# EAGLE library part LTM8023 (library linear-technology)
2A, 36V DC/DC µModule Complete Step-Down Switch Mode Power Supply Source: http://www.linear.com/pc/downloadDocument.do?name=8023ff.pdf
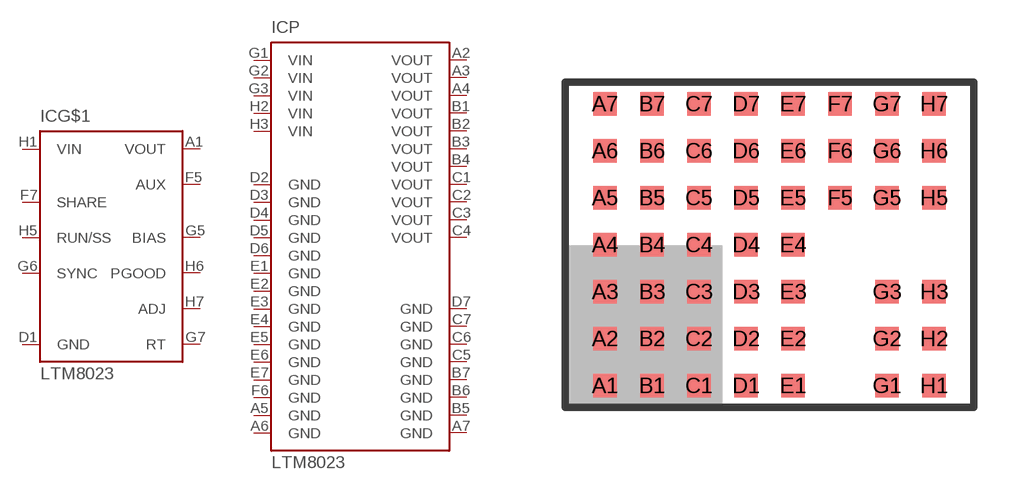
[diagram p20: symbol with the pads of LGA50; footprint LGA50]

Designator prefix IC; gates G$1=LTM8023 P=LTM8023-P

## LTM8023 (MPN: LTM8023IV#PBF; OC_FARNELL: 1799827; OC_NEWARK: 02P7640)  [LGA50]
A1  G$1:VOUT  pwr
A2  P:VOUT  pwr
A3  P:VOUT  pwr
A4  P:VOUT  pwr
A5  P:GND  pwr
A6  P:GND  pwr
A7  P:GND  pwr
B1  P:VOUT  pwr
B2  P:VOUT  pwr
B3  P:VOUT  pwr
B4  P:VOUT  pwr
B5  P:GND  pwr
B6  P:GND  pwr
B7  P:GND  pwr
C1  P:VOUT  pwr
C2  P:VOUT  pwr
C3  P:VOUT  pwr
C4  P:VOUT  pwr
C5  P:GND  pwr
C6  P:GND  pwr
C7  P:GND  pwr
D1  G$1:GND  pwr
D2  P:GND  pwr
D3  P:GND  pwr
D4  P:GND  pwr
D5  P:GND  pwr
D6  P:GND  pwr
D7  P:GND  pwr
E1  P:GND  pwr
E2  P:GND  pwr
E3  P:GND  pwr
E4  P:GND  pwr
E5  P:GND  pwr
E6  P:GND  pwr
E7  P:GND  pwr
F5  G$1:AUX  out
F6  P:GND  pwr
F7  G$1:SHARE  in
G1  P:VIN  pwr
G2  P:VIN  pwr
G3  P:VIN  pwr
G5  G$1:BIAS  pas
G6  G$1:SYNC  in
G7  G$1:RT  pas
H1  G$1:VIN  pwr
H2  P:VIN  pwr
H3  P:VIN  pwr
H5  G$1:RUN/SS  in
H6  G$1:PGOOD  oc
H7  G$1:ADJ  pas

## Footprint LGA50 (pad centres in mm)
LGA Package 50-Lead (11.25mm × 9.00mm × 2.82mm) (Reference LTC DWG # 05-08-1804 Rev B) Source: http://www.linear.com/pc/downloadDocument.do?name=8023ff.pdf
smd 0.635 x 0.635: A1 -4.445,-3.81; A2 -4.445,-2.54; A3 -4.445,-1.27; A4 -4.445,0; A5 -4.445,1.27; A6 -4.445,2.54; A7 -4.445,3.81; B1 -3.175,-3.81; B2 -3.175,-2.54; B3 -3.175,-1.27; B4 -3.175,0; B5 -3.175,1.27; B6 -3.175,2.54; B7 -3.175,3.81; C1 -1.905,-3.81; C2 -1.905,-2.54; C3 -1.905,-1.27; C4 -1.905,0; C5 -1.905,1.27; C6 -1.905,2.54; C7 -1.905,3.81; D1 -0.635,-3.81; D2 -0.635,-2.54; D3 -0.635,-1.27; D4 -0.635,0; D5 -0.635,1.27; D6 -0.635,2.54; D7 -0.635,3.81; E1 0.635,-3.81; E2 0.635,-2.54; E3 0.635,-1.27; E4 0.635,0; E5 0.635,1.27; E6 0.635,2.54; E7 0.635,3.81; F5 1.905,1.27; F6 1.905,2.54; F7 1.905,3.81; G1 3.175,-3.81; G2 3.175,-2.54; G3 3.175,-1.27; G5 3.175,1.27; G6 3.175,2.54; G7 3.175,3.81; H1 4.445,-3.81; H2 4.445,-2.54; H3 4.445,-1.27; H5 4.445,1.27; H6 4.445,2.54; H7 4.445,3.81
